(* Logix 5000 AddOnInstructionDefinition export AMCI_MSO_and_Preset_to_Absolute_Encoder; software revision 20.05 *)

TYPE AMCI_Motion_Axis_Output_Data :
STRUCT
   Control_Word_0 : INT;
   Control_Word_1 : INT;
   Position_or_Distance : DINT;
   Programmed_Speed : DINT;
   Acceleration : INT;
   Deceleration : INT;
   Output_Word_8 : INT;
   Output_Word_9 : INT;
END_STRUCT
END_TYPE

TYPE AMCI_Motion_Axis_Input_Data :
STRUCT
   Moving_CW : BOOL;
   Moving_CCW : BOOL;
   In_Hold_State : BOOL;
   Stopped : BOOL;
   At_Home : BOOL;
   Accelerating : BOOL;
   Decelerating : BOOL;
   Move_Complete : BOOL;
   Status_Word_0_Bit_8 : BOOL;
   Status_Word_0_Bit_9 : BOOL;
   Position_Invalid : BOOL;
   Input_Error : BOOL;
   Command_Error : BOOL;
   Configuration_Error : BOOL;
   Module_OK : BOOL;
   Mode_Flag : BOOL;
   IN1_Active : BOOL;
   IN2_Active : BOOL;
   IN3_Active : BOOL;
   IN4_Active : BOOL;
   Status_Word_1_Bit_4 : BOOL;
   Status_Word_1_Bit_5 : BOOL;
   Connection_Was_Lost : BOOL;
   Driver_Fault : BOOL;
   Status_Word_1_Bit_8 : BOOL;
   Invalid_Jog_Change : BOOL;
   Status_Word_1_Bit_10 : BOOL;
   Heartbeat_Bit : BOOL;
   Status_Word_1_Bit_12 : BOOL;
   Status_Word_1_Bit_13 : BOOL;
   Stall_Detected : BOOL;
   Drive_Is_Enabled : BOOL;
   Motor_Position : DINT;
   Encoder_Position : DINT;
   Trapped_Encoder_Position : DINT;
   Input_Word_8 : INT;
   Input_Word_9 : INT;
END_STRUCT
END_TYPE

ADD_ON_INSTRUCTION AMCI_MSO_and_Preset_to_Absolute_Encoder   (* revision 2.0, vendor AMCI, ExecuteEnableInFalse *)
// Enables and sets the motor position to the absolute encoder position.   Only for AMCI SMDXXE2 with Absolute Encoders.
// Revision note:
// 3/8/23: Revision 2.  Changed the name to MSO and Preset to Absolute Encoder.   No change the functionality.
// Help:
// This AOI will only work with SMDXXE2 units with an absolute encoder.  This AOI WILL NOT WORK with SDXXXXXE2 or SVXXXE2 units.
// This instruction enables the motion device before presetting the motor position to the absolute encoder position.
// AXIS INPUT DATA:  Input data from AMCI motion device.   Uses the AMCI_Motion_Axis_Input_Data User Defined Data Type.
// AXIS OUTPUT DATA; Output data from the AOI to the AMCI motion device.   Uses the AMCI_Motion_Axis_Output_Data User Defined Data Type.
// EN (Enable) Set when rung is true, Reset when rung is false
// DN (Done) Set when command is sent to the motion device.  Reset when the rung is false.
// ER (Error) Set when a command or input error failed to clear.  Reset when the rung is false.
VAR_IN_OUT
   Axis_Input_Data : AMCI_Motion_Axis_Input_Data; {required}
        [0].6   // set when decelerating
   Axis_Output_Data : AMCI_Motion_Axis_Output_Data; {required}
END_VAR
VAR_OUTPUT
   EN : BOOL; {visible}   // set when rung with AOI is true
   DN : BOOL; {access Read Only, visible}   // set when preset motor position command sent to motion axis
   ER : BOOL; {access Read Only, visible}   // set when input, command, or configuraiton error
END_VAR
VAR
   command_data_block : INT[10];
        [0]   // Command Bits MSW
        [1]   // Command Bits LSW
        [2]   // Upper Target Position
        [3]   // Lower Target Position
        [4]   // Upper Programmed Speed
        [5]   // Lower Programmed Speed
   enable_timer : TIMER := (PRE := 100); {access None}
   driver_enabled : DINT; {access None}
END_VAR

ROUTINE EnableInFalse   (* ladder *)
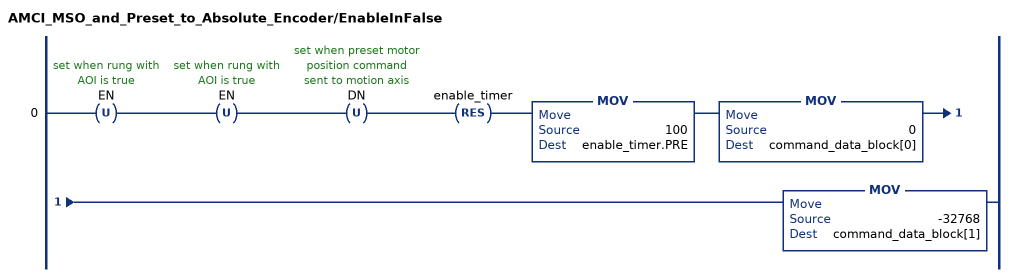
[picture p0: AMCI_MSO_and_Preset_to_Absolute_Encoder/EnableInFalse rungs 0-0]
   0: OTU(EN)OTU(EN)OTU(DN)RES(enable_timer)MOV(100,enable_timer.PRE)MOV(0,command_data_block[0])MOV(-32768,command_data_block[1]);
END_ROUTINE

ROUTINE Logic   (* ladder *)
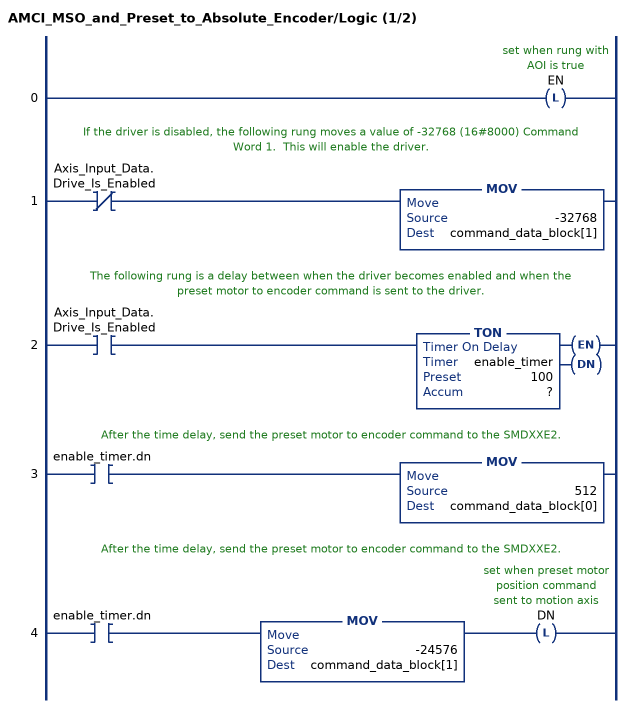
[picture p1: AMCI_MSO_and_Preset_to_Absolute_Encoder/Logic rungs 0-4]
   0: OTL(EN);
   // If the driver is disabled, the following rung moves a value of -32768 (16#8000) Command Word 1.  This will enable the driver.
   1: XIO(Axis_Input_Data.Drive_Is_Enabled)MOV(-32768,command_data_block[1]);
   // The following rung is a delay between when the driver becomes enabled and when the preset motor to encoder command is sent to the driver.
   2: XIC(Axis_Input_Data.Drive_Is_Enabled)TON(enable_timer,?,?);
   // After the time delay, send the preset motor to encoder command to the SMDXXE2.
   3: XIC(enable_timer.dn)MOV(512,command_data_block[0]);
   // After the time delay, send the preset motor to encoder command to the SMDXXE2.
   4: XIC(enable_timer.dn)MOV(-24576,command_data_block[1])OTL(DN);
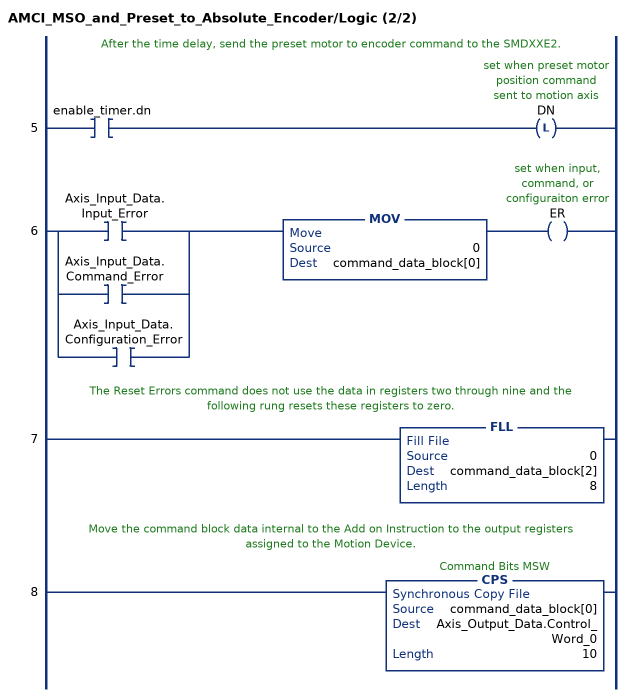
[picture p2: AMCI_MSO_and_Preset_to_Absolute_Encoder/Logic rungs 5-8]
   // After the time delay, send the preset motor to encoder command to the SMDXXE2.
   5: XIC(enable_timer.dn)OTL(DN);
   6: [XIC(Axis_Input_Data.Input_Error) ,XIC(Axis_Input_Data.Command_Error) ,XIC(Axis_Input_Data.Configuration_Error) ]MOV(0,command_data_block[0])OTE(ER);
   // The Reset Errors command does not use the data in registers two through nine and the following rung resets these registers to zero.
   7: FLL(0,command_data_block[2],8);
   // Move the command block data internal to the Add on Instruction to the output registers assigned to the Motion Device.
   8: CPS(command_data_block[0],Axis_Output_Data.Control_Word_0,10);
END_ROUTINE
END_ADD_ON_INSTRUCTION
